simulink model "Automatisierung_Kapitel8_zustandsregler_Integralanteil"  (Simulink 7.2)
settings: Solver=ode45  StartTime=0.0  StopTime=100  MaxStep=0.2  RelTol=1e-3
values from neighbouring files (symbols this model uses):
  Ac = [0,1,0,0;-1,-1,1,1;0,0,0,1;0.1,0.1,-0.2,-0.2]    [Automatisierung_Kapitel8.m]
  Bc = [bc,bvc]    [Automatisierung_Kapitel8.m]
  Cc = eye(4)    [Automatisierung_Kapitel8.m]
  Dc = [0,0;0,0;0,0;0,0]    [Automatisierung_Kapitel8.m]
  kI = ke(5)    [Automatisierung_Kapitel8.m]
  kP = 1/(cc*inv(eye(4)-Ad)*bd)    [Automatisierung_Kapitel8.m]
  kx = kP*cc+ke(1:4)    [Automatisierung_Kapitel8.m]
  Ta = 2    [Automatisierung_Kapitel8.m]
libraries: simulink x1

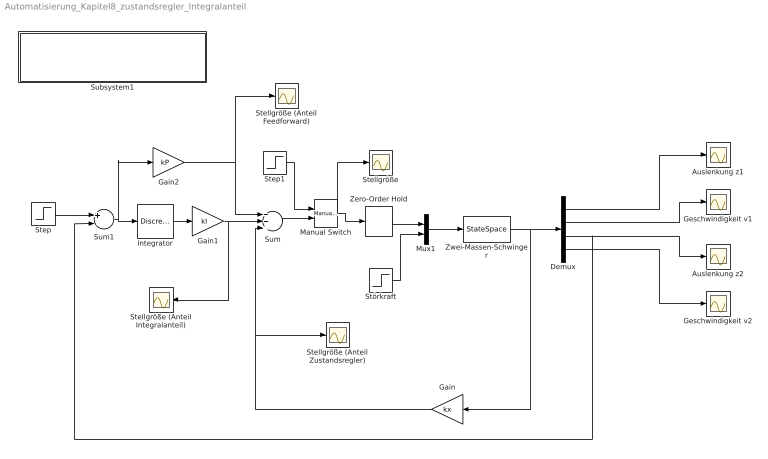
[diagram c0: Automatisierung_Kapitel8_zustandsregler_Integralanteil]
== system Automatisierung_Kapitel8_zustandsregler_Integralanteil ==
  Auslenkung z1 : Scope
  Auslenkung z2 : Scope
  Demux : Demux
  Gain : Gain  Orientation=left  Gain=kx  Multiplication=Matrix(K*u)  ParameterDataType=sfix(16)  ParameterScaling=2^0  OutDataType=sfix(16)  OutScaling=2^0  SampleTime=Ta
  Gain1 : Gain  Gain=kI  ParameterDataType=sfix(16)  ParameterScaling=2^0  OutDataType=sfix(16)  OutScaling=2^0
  Gain2 : Gain  Gain=kP  ParameterDataType=sfix(16)  ParameterScaling=2^0  OutDataType=sfix(16)  OutScaling=2^0
  Geschwindigkeit v1 : Scope
  Geschwindigkeit v2 : Scope
  Integrator : DiscreteTransferFcn  Denominator=[1 -1]  SampleTime=Ta
  Manual Switch : simulink/Signal Routing/Manual Switch  SystemSampleTime=-1  sw=0  action=0  varsize=off
  Mux1 : Mux  Inputs=2
  Stellgröße : Scope
  Stellgröße (Anteil Feedforward) : Scope
  Stellgröße (Anteil Integralanteil) : Scope
  Stellgröße (Anteil Zustandsregler) : Scope
  Step : Step  Time=0  SampleTime=Ta
  Step1 : Step  Time=0  SampleTime=0
  Störkraft : Step  Time=20  SampleTime=0
  Subsystem1 : Subsystem
  Sum : Sum  Inputs=+++  OutDataType=sfix(16)  OutScaling=2^0
  Sum1 : Sum  Inputs=+-  OutDataType=sfix(16)  OutScaling=2^0  SampleTime=Ta
  Zero-Order Hold : ZeroOrderHold  SampleTime=Ta
  Zwei-Massen-Schwinger : StateSpace  A=Ac  B=Bc  C=Cc  D=Dc  X0=[0,0,0,0]
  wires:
  Zwei-Massen-Schwinger/1 -> Demux/1, Gain/1
  Mux1/1 -> Zwei-Massen-Schwinger/1
  Zero-Order Hold/1 -> Mux1/1
  Störkraft/1 -> Mux1/2
  Demux/1 -> Auslenkung z1/1
  Demux/3 -> Auslenkung z2/1, Sum1/2
  Demux/2 -> Geschwindigkeit v1/1
  Demux/4 -> Geschwindigkeit v2/1
  Gain2/1 -> Sum/1, Stellgröße (Anteil Feedforward)/1
  Sum/1 -> Manual Switch/2
  Manual Switch/1 -> Zero-Order Hold/1, Stellgröße/1
  Step1/1 -> Manual Switch/1
  Step/1 -> Sum1/1
  Sum1/1 -> Integrator/1, Gain2/1
  Gain/1 -> Sum/3, Stellgröße (Anteil Zustandsregler)/1
  Integrator/1 -> Gain1/1
  Gain1/1 -> Sum/2, Stellgröße (Anteil Integralanteil)/1

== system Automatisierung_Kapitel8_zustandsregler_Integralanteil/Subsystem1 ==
